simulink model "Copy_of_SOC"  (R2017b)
settings: Solver=FixedStepDiscrete  StartTime=0.0  StopTime=10.0  FixedStep=0.01  RelTol=1e-3  EnableMultiTasking=on
undefined symbols (not defined in the file): ASWTYPE_FALSE, ASWTYPE_TRUE, CaSOC_OneSOCVoltTable_mV, CaSOC_ZeroSOCTempTable_C, CaSOC_ZeroSOCVoltTable_mV, CbSOC_ManualDeplaCorrect_flg, CbSOC_ManuOCVCorrect_flg, CbSOC_SOCHighDiagOn_flg, CbSOC_SOCLowDiagOn_flg, CcSOC_ACChrgFinishDispSOC_pct, CcSOC_ACChrgFinishMaxSOC_pct, CcSOC_ACStepChrgMaxSOC_pct, CcSOC_AllowMaxCellSOC_pct, CcSOC_AllowMinCellSOC_pct, CcSOC_CapCalcCycl_ms, CcSOC_CellMinTempFilterAvg_numb, CcSOC_CellVoltMeasTol_mV, CcSOC_ChrgFishBefMaxSOC_pct, CcSOC_ChrgFishBefMinSOC_pct, CcSOC_ChrgFollowCurr_A, CcSOC_DCChrgFinishDispSOC_pct, CcSOC_DCChrgFinishMaxSOC_pct, CcSOC_DCStepChrgMaxSOC_pct, CcSOC_DeplaCellVoltMeasTol_mV, CcSOC_DeplaCorrectSOCDiff_pct, CcSOC_DisChrgFlwCurr_A, CcSOC_DispSOCChgSleepTime_min, CcSOC_DispSOCCordRunTi_ms, CcSOC_DispSOCErr_pct, CcSOC_FlwTarSOCDiff_pct, CcSOC_FullChrgTempThrld_C, CcSOC_MaxFlwDispSOC_pct, CcSOC_MinFlwDispSOC_pct, CcSOC_OCVCorrectRunTime_ms, CcSOC_OCVCorrectSleepTime_min, CcSOC_OCVCorrectSOCDiff_pct, CcSOC_OCVPeakCellVoltDev_mV, CcSOC_OCVPeakCellVoltTime_ms, CcSOC_PackSOCUseMax_pct, CcSOC_PackSOCUseMin_pct, CcSOC_SOCDeplaCurrThrd_A, CcSOC_SOCDeplaCurrThrdTi_ms, CcSOC_SOCDeplaNoOCVTi_min, CcSOC_SOCDeplaOCVTi_min, CcSOC_SOCHighAlarmThrld_pct, CcSOC_SOCHighWarningThrld_pct, CcSOC_SOCHysValue_pct, CcSOC_SOCLowAlarmThrld_pct, CcSOC_SOCLowWarningThrld_pct, CcSOC_ZeroMinSOC_pct, CcSOC_ZeroPackCrntThrd_A, CcSOC_ZeroSOCRunTime_ms, Enum_CTCCtrCtlConnMode, Enum_MSMBMUState, SOC_CONST0_NUMB, SOC_CONST1000_NUMB, SOC_CONST100_NUMB, SOC_CONST2080_NUMB, SOC_CONST3600000_NUMB, SOC_CONST60000_NUMB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
libraries: AIWAYS_Powertrain_BMS_lib x109
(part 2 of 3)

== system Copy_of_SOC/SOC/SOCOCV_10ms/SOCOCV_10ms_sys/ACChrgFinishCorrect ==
  LcCDP_MinCellAvgFitTemp_C : Inport
  Enable : EnablePort
  Constant1 : Constant  Value=CcSOC_ACChrgFinishDispSOC_pct
  Constant2 : Constant  Value=CcSOC_FullChrgTempThrld_C
  Data Store Write2 : AIWAYS_Powertrain_BMS_lib/Signals/Data Store Write  Priority=0  DSW=EcNVM_DispSOC_pct
  MaxMinSOCCorrect : Subsystem  TreatAsAtomicUnit=on
  Relational Operator : RelationalOperator  OutDataTypeStr=boolean
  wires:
  Relational Operator/1 -> MaxMinSOCCorrect/Enable
  Constant2/1 -> Relational Operator/2
  LcCDP_MinCellAvgFitTemp_C/1 -> Relational Operator/1
  Constant1/1 -> Data Store Write2/1

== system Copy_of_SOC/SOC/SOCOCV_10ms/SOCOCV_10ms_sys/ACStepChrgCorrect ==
  Enable : EnablePort
  Add : Sum  Inputs=+-  AccumDataTypeStr=single  OutDataTypeStr=single
  Add1 : Sum  Inputs=+-  AccumDataTypeStr=single  OutDataTypeStr=single
  Constant : Constant  Value=CcSOC_ACStepChrgMaxSOC_pct
  Constant1 : Constant  Value=CcSOC_ACStepChrgMaxSOC_pct
  Constant2 : Constant  Value=SOC_CONST100_NUMB
  Constant3 : Constant  Value=SOC_CONST0_NUMB
  Data Store Read : AIWAYS_Powertrain_BMS_lib/Signals/Data Store Read  Priority=0  DSR=EcNVM_MinCellSOC_pct
  Data Store Read1 : AIWAYS_Powertrain_BMS_lib/Signals/Data Store Read  Priority=0  DSR=EcNVM_MaxCellSOC_pct
  Data Store Write : AIWAYS_Powertrain_BMS_lib/Signals/Data Store Write  DSW=EcNVM_MaxCellSOC_pct
  Data Store Write1 : AIWAYS_Powertrain_BMS_lib/Signals/Data Store Write  DSW=EcNVM_MinCellSOC_pct
  Limiter : AIWAYS_Powertrain_BMS_lib/Nonlinear Blocks/Limiter
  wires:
  Constant/1 -> Data Store Write/1
  Data Store Read/1 -> Add/1
  Data Store Read1/1 -> Add1/1
  Constant1/1 -> Add1/2
  Add1/1 -> Add/2
  Limiter/1 -> Data Store Write1/1
  Constant2/1 -> Limiter/1
  Constant3/1 -> Limiter/2
  Add/1 -> Limiter/3

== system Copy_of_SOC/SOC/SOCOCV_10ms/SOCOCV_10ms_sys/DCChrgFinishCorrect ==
  LcCDP_MinCellAvgFitTemp_C : Inport
  Enable : EnablePort
  Constant1 : Constant  Value=CcSOC_DCChrgFinishDispSOC_pct
  Constant2 : Constant  Value=CcSOC_FullChrgTempThrld_C
  Data Store Write1 : AIWAYS_Powertrain_BMS_lib/Signals/Data Store Write  DSW=EcNVM_DispSOC_pct
  MaxMinSOCCorrect : Subsystem  TreatAsAtomicUnit=on
  Relational Operator : RelationalOperator  OutDataTypeStr=boolean
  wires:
  Relational Operator/1 -> MaxMinSOCCorrect/Enable
  Constant2/1 -> Relational Operator/2
  LcCDP_MinCellAvgFitTemp_C/1 -> Relational Operator/1
  Constant1/1 -> Data Store Write1/1

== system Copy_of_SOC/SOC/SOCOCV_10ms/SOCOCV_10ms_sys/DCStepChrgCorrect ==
  Enable : EnablePort
  Add : Sum  Inputs=+-  AccumDataTypeStr=single  OutDataTypeStr=single
  Add1 : Sum  Inputs=+-  AccumDataTypeStr=single  OutDataTypeStr=single
  Constant : Constant  Value=CcSOC_DCStepChrgMaxSOC_pct
  Constant1 : Constant  Value=CcSOC_DCStepChrgMaxSOC_pct
  Constant2 : Constant  Value=SOC_CONST100_NUMB
  Constant3 : Constant  Value=SOC_CONST0_NUMB
  Data Store Read : AIWAYS_Powertrain_BMS_lib/Signals/Data Store Read  Priority=0  DSR=EcNVM_MinCellSOC_pct
  Data Store Read1 : AIWAYS_Powertrain_BMS_lib/Signals/Data Store Read  Priority=0  DSR=EcNVM_MaxCellSOC_pct
  Data Store Write : AIWAYS_Powertrain_BMS_lib/Signals/Data Store Write  DSW=EcNVM_MaxCellSOC_pct
  Data Store Write1 : AIWAYS_Powertrain_BMS_lib/Signals/Data Store Write  DSW=EcNVM_MinCellSOC_pct
  Limiter : AIWAYS_Powertrain_BMS_lib/Nonlinear Blocks/Limiter
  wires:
  Limiter/1 -> Data Store Write1/1
  Add/1 -> Limiter/3
  Add1/1 -> Add/2
  Constant1/1 -> Add1/2
  Data Store Read1/1 -> Add1/1
  Data Store Read/1 -> Add/1
  Constant/1 -> Data Store Write/1
  Constant2/1 -> Limiter/1
  Constant3/1 -> Limiter/2

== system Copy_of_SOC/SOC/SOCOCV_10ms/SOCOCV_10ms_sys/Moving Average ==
  note: Moving Average
  u : Inport
  R : Inport  Port=2  OutDataTypeStr=boolean
  Chart : Stateflow chart  TreatAsAtomicUnit=on
  Signal Conversion : SignalConversion  ConversionOutput=Contiguous copy  OverrideOpt=off
  y : Outport
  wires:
  Signal Conversion/1 -> y/1
  Chart/1(Y) -> Signal Conversion/1
  u/1 -> Chart/1(u)
  R/1 -> Chart/2(R)

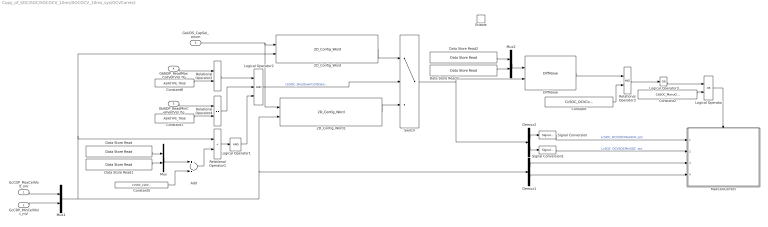
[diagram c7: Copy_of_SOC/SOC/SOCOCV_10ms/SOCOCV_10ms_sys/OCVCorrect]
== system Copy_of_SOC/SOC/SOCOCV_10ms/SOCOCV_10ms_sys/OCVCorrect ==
  GcCDP_MaxCellVolt_mV : Inport
  GcCDP_MinCellVolt_mV : Inport  Port=2
  GeUDS_CapSel_enum : Inport  Port=3
  GbNDP_ReadMaxCellVoltVld_flg : Inport  Port=4
  GbNDP_ReadMinCellVoltVld_flg : Inport  Port=5
  Enable : EnablePort
  2D_Config_Word : AIWAYS_Powertrain_BMS_lib/Signals/2D_Config_Word  Default_Cal_Breakpoint1_Name=CaSOC_CATL203ChrgOCVSOCCellVolt_mV  Default_Cal_Table1_Name=CaSOC_CATL203ChrgOCVSOCCellSOC_pct  CATL153Ah_Cal_Breakpoint1_Name=CaSOC_TFE177ChrgOCVSOCCellVolt_mV  CATL153Ah_Cal_Table1_Name=CaSOC_TFE177ChrgOCVSOCCellSOC_pct  CATL180Ah_Cal_Breakpoint1_Name=CaSOC_TFE177ChrgOCVSOCCellVolt_mV  CATL180Ah_Cal_Table1_Name=CaSOC_TFE177ChrgOCVSOCCellSOC_pct  CATL177Ah_Cal_Breakpoint1_Name=CaSOC_CATL177ChrgOCVSOCCellVolt_mV  CATL177Ah_Cal_Table1_Name=CaSOC_CATL177ChrgOCVSOCCellSOC_pct  CATL203Ah_Cal_Breakpoint1_Name=CaSOC_CATL203ChrgOCVSOCCellVolt_mV  CATL203Ah_Cal_Table1_Name=CaSOC_CATL203ChrgOCVSOCCellSOC_pct  CATL51Ah_Cal_Breakpoint1_Name=CaSOC_TFE177ChrgOCVSOCCellVolt_mV  CATL51Ah_Cal_Table1_Name=CaSOC_TFE177ChrgOCVSOCCellSOC_pct  CATL132Ah_Cal_Breakpoint1_Name=CaSOC_TFE177ChrgOCVSOCCellVolt_mV  CATL132Ah_Cal_Table1_Name=CaSOC_TFE177ChrgOCVSOCCellSOC_pct  XWD75Ah_Cal_Breakpoint1_Name=CaSOC_XWD75ChrgOCVSOCCellVolt_mV  XWD75Ah_Cal_Table1_Name=CaSOC_XWD75ChrgOCVSOCCellSOC_pct  TFE177Ah_Cal_Breakpoint1_Name=CaSOC_TFE177ChrgOCVSOCCellVolt_mV  TFE177Ah_Cal_Table1_Name=CaSOC_TFE177ChrgOCVSOCCellSOC_pct  CATLCTP248Ah_Cal_Breakpoint1_Name=CaSOC_TFE177ChrgOCVSOCCellVolt_mV  CATLCTP248Ah_Cal_Table1_Name=CaSOC_TFE177ChrgOCVSOCCellSOC_pct
  2D_Config_Word1 : AIWAYS_Powertrain_BMS_lib/Signals/2D_Config_Word  Default_Cal_Breakpoint1_Name=CaSOC_CATL203DisChrgOCVSOCCellVolt_mV  Default_Cal_Table1_Name=CaSOC_CATL203DisChrgOCVSOCCellSOC_pct  CATL153Ah_Cal_Breakpoint1_Name=CaSOC_TFE177DisChrgOCVSOCCellVolt_mV  CATL153Ah_Cal_Table1_Name=CaSOC_TFE177DisChrgOCVSOCCellSOC_pct  CATL180Ah_Cal_Breakpoint1_Name=CaSOC_TFE177DisChrgOCVSOCCellVolt_mV  CATL180Ah_Cal_Table1_Name=CaSOC_TFE177DisChrgOCVSOCCellSOC_pct  CATL177Ah_Cal_Breakpoint1_Name=CaSOC_CATL177DisChrgOCVSOCCellVolt_mV  CATL177Ah_Cal_Table1_Name=CaSOC_CATL177DisChrgOCVSOCCellSOC_pct  CATL203Ah_Cal_Breakpoint1_Name=CaSOC_CATL203DisChrgOCVSOCCellVolt_mV  CATL203Ah_Cal_Table1_Name=CaSOC_CATL203DisChrgOCVSOCCellSOC_pct  CATL51Ah_Cal_Breakpoint1_Name=CaSOC_TFE177DisChrgOCVSOCCellVolt_mV  CATL51Ah_Cal_Table1_Name=CaSOC_TFE177DisChrgOCVSOCCellSOC_pct  CATL132Ah_Cal_Breakpoint1_Name=CaSOC_TFE177DisChrgOCVSOCCellVolt_mV  CATL132Ah_Cal_Table1_Name=CaSOC_TFE177DisChrgOCVSOCCellSOC_pct  XWD75Ah_Cal_Breakpoint1_Name=CaSOC_XWD75DisChrgOCVSOCCellVolt_mV  XWD75Ah_Cal_Table1_Name=CaSOC_XWD75DisChrgOCVSOCCellSOC_pct  TFE177Ah_Cal_Breakpoint1_Name=CaSOC_TFE177DisChrgOCVSOCCellVolt_mV  TFE177Ah_Cal_Table1_Name=CaSOC_TFE177DisChrgOCVSOCCellSOC_pct  CATLCTP248Ah_Cal_Breakpoint1_Name=CaSOC_TFE177DisChrgOCVSOCCellVolt_mV  CATLCTP248Ah_Cal_Table1_Name=CaSOC_TFE177DisChrgOCVSOCCellSOC_pct
  Add : Sum  Inputs=+-  AccumDataTypeStr=uint16  OutDataTypeStr=uint16
  Constant : Constant  Value=CcSOC_OCVCorrectSOCDiff_pct
  Constant1 : Constant  Value=ASWTYPE_TRUE
  Constant2 : Constant  Value=CbSOC_ManuOCVCorrect_flg
  Constant5 : Constant  Value=CcSOC_CellVoltMeasTol_mV
  Constant6 : Constant  Value=ASWTYPE_TRUE
  Data Store Read : AIWAYS_Powertrain_BMS_lib/Signals/Data Store Read  Priority=0  DSR=EcNVM_MaxCellVolt_mV
  Data Store Read1 : AIWAYS_Powertrain_BMS_lib/Signals/Data Store Read  Priority=0  DSR=EcNVM_MinCellVolt_mV
  Data Store Read2 : AIWAYS_Powertrain_BMS_lib/Signals/Data Store Read  Priority=0  DSR=EcNVM_MaxCellSOC_pct
  Data Store Read3 : AIWAYS_Powertrain_BMS_lib/Signals/Data Store Read  Priority=0  DSR=EcNVM_MinCellSOC_pct
  Demux1 : Demux  Outputs=2
  Demux2 : Demux  Outputs=2
  DiffValue : AIWAYS_Powertrain_BMS_lib/Mathematical Functions/DiffValue
  Logical Operator : Logic  Operator=OR  AllPortsSameDT=off  OutDataTypeStr=boolean
  Logical Operator1 : Logic  Inputs=1  AllPortsSameDT=off  OutDataTypeStr=boolean
  Logical Operator2 : Logic  Inputs=3  AllPortsSameDT=off  OutDataTypeStr=boolean
  Logical Operator3 : Logic  Operator=OR  Inputs=1  AllPortsSameDT=off  OutDataTypeStr=boolean
  MaxCellCorrect : Subsystem  TreatAsAtomicUnit=on
  Mux : Mux  Inputs=2
  Mux1 : Mux  Inputs=2
  Mux2 : Mux  Inputs=2
  Relational Operator1 : RelationalOperator  Operator=<  OutDataTypeStr=boolean
  Relational Operator2 : RelationalOperator  Operator===  OutDataTypeStr=boolean
  Relational Operator3 : RelationalOperator  OutDataTypeStr=boolean
  Relational Operator4 : RelationalOperator  Operator===  OutDataTypeStr=boolean
  Signal Conversion : SignalConversion  OverrideOpt=off
  Signal Conversion1 : SignalConversion  OverrideOpt=off
  Switch : Switch  Criteria=u2 ~= 0
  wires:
  Logical Operator3/1 -> Logical Operator/1
  Constant2/1 -> Logical Operator/2
  Signal Conversion/1 -> MaxCellCorrect/1(LcSOC_OCVSOCMaxSOC_pct)  "LcSOC_OCVSOCMaxSOC_pct"
  Logical Operator/1 -> MaxCellCorrect/Enable
  Relational Operator3/1 -> Logical Operator3/1
  Data Store Read1/1 -> Mux/2
  Data Store Read/1 -> Mux/1
  GcCDP_MinCellVolt_mV/1 -> Mux1/2
  GcCDP_MaxCellVolt_mV/1 -> Mux1/1
  Mux1/1 -> 2D_Config_Word/2, Relational Operator1/1, 2D_Config_Word1/2, Demux1/1
  Relational Operator1/1 -> Logical Operator1/1
  Mux/1 -> Add/1
  Constant5/1 -> Add/2
  Constant6/1 -> Relational Operator2/2
  GbNDP_ReadMaxCellVoltVld_flg/1 -> Relational Operator2/1
  GbNDP_ReadMinCellVoltVld_flg/1 -> Relational Operator4/1
  Constant1/1 -> Relational Operator4/2
  Relational Operator2/1 -> Logical Operator2/1
  Relational Operator4/1 -> Logical Operator2/2
  Add/1 -> Relational Operator1/2
  Data Store Read2/1 -> Mux2/1
  Data Store Read3/1 -> Mux2/2
  DiffValue/1 -> Relational Operator3/1
  Constant/1 -> Relational Operator3/2
  Mux2/1 -> DiffValue/1
  Demux2/1 -> Signal Conversion/1
  Demux2/2 -> Signal Conversion1/1
  Signal Conversion1/1 -> MaxCellCorrect/2(LcSOC_OCVSOCMinSOC_pct)  "LcSOC_OCVSOCMinSOC_pct"
  Logical Operator2/1 -> Switch/2  "LbSOC_ShutdownCellState_flg"
  2D_Config_Word/1 -> Switch/1
  2D_Config_Word1/1 -> Switch/3
  Switch/1 -> DiffValue/2, Demux2/1
  Logical Operator1/1 -> Logical Operator2/3
  Demux1/1 -> MaxCellCorrect/3(GcCDP_MaxCellVolt_mV)
  Demux1/2 -> MaxCellCorrect/4(GcCDP_MinCellVolt_mV)
  GeUDS_CapSel_enum/1 -> 2D_Config_Word1/1, 2D_Config_Word/1

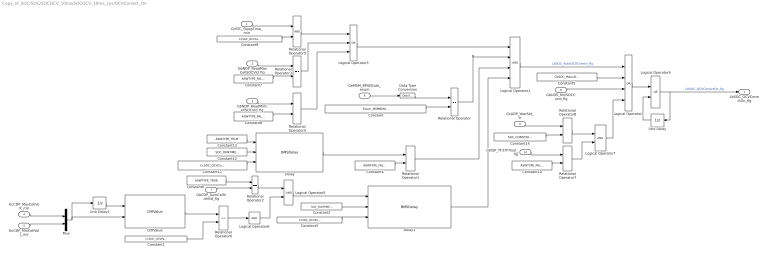
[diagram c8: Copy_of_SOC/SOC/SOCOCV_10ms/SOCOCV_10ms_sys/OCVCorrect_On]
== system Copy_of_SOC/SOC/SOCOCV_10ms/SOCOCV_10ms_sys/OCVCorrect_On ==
  GcRTC_SleepTime_min : Inport
  GbNDP_ReadMaxCellSOCVld_flg : Inport  Port=2
  GbNDP_ReadMinCellSOCVld_flg : Inport  Port=3
  GcCDP_MaxCellVolt_mV : Inport  Port=4
  GcCDP_MinCellVolt_mV : Inport  Port=5
  GeMSM_BMUState_enum : Inport  Port=6
  GbCDP_SumCellVoltVld_flg : Inport  Port=7
  GbUDS_MnlSOCCorrd_flg : Inport  Port=8
  GcADP_YearSet_Yr : Inport  Port=9
  GbISP_TF37FTiout_flg : Inport  Port=10
  Constant : Constant  Value=Enum_MSMBMUState.Enum_MSMBMUState_Standby
  Constant1 : Constant  Value=CcSOC_OCVPeakCellVoltDev_mV
  Constant{4,7..8,10} (4 alike) : Constant  Value=ASWTYPE_FALSE
  Constant11 : Constant  Value=CcSOC_OCVCorrectRunTime_ms
  Constant12 : Constant  Value=SOC_RUNTIME_MS
  Constant13 : Constant  Value=ASWTYPE_TRUE
  Constant14 : Constant  Value=SOC_CONST2080_NUMB
  Constant2 : Constant  Value=SOC_RUNTIME_MS
  Constant3 : Constant  Value=CcSOC_OCVPeakCellVoltTime_ms
  Constant5 : Constant  Value=CbSOC_ManuOCVCorrect_flg
  Constant6 : Constant  Value=ASWTYPE_TRUE
  Constant9 : Constant  Value=CcSOC_OCVCorrectSleepTime_min
  Data Type Conversion : DataTypeConversion
  Delay : AIWAYS_Powertrain_BMS_lib/Debounce & Delay/BMSDelay
  Delay1 : AIWAYS_Powertrain_BMS_lib/Debounce & Delay/BMSDelay
  DiffValue : AIWAYS_Powertrain_BMS_lib/Mathematical Functions/DiffValue
  Logical Operator1 : Logic  Inputs=4  AllPortsSameDT=off  OutDataTypeStr=boolean
  Logical Operator2 : Logic  Operator=OR  Inputs=4  AllPortsSameDT=off  OutDataTypeStr=boolean
  Logical Operator3 : Logic  Operator=OR  Inputs=3  AllPortsSameDT=off  OutDataTypeStr=boolean
  Logical Operator4 : Logic  Operator=OR  AllPortsSameDT=off  OutDataTypeStr=boolean
  Logical Operator5 : Logic  AllPortsSameDT=off  OutDataTypeStr=boolean
  Logical Operator6 : Logic  Inputs=1  AllPortsSameDT=off  OutDataTypeStr=boolean
  Logical Operator7 : Logic  AllPortsSameDT=off  OutDataTypeStr=boolean
  Mux : Mux  Inputs=2
  Relational Operator{,1..4,7..8} (7 alike) : RelationalOperator  Operator===  OutDataTypeStr=boolean
  Relational Operator5 : RelationalOperator  OutDataTypeStr=boolean
  Relational Operator6 : RelationalOperator  Operator=<=  OutDataTypeStr=boolean
  Unit Delay : UnitDelay  SampleTime=-1  StateName=StateName
  Unit Delay1 : UnitDelay  SampleTime=-1  StateName=StateName
  LbSOC_OCVCorrectOn_flg : Outport
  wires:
  Constant12/1 -> Delay/2
  Relational Operator6/1 -> Logical Operator6/1
  Delay/1 -> Relational Operator1/1
  Constant7/1 -> Relational Operator3/2
  Logical Operator6/1 -> Logical Operator5/2
  Mux/1 -> Unit Delay1/1, DiffValue/2
  GbNDP_ReadMinCellSOCVld_flg/1 -> Relational Operator4/1
  Constant9/1 -> Relational Operator5/2
  Constant1/1 -> Relational Operator6/2
  Logical Operator4/1 -> LbSOC_OCVCorrectOn_flg/1, Unit Delay/1  "LbSOC_OCVCorrectOn_flg"
  Logical Operator5/1 -> Delay1/1
  Data Type Conversion/1 -> Relational Operator/1
  GcCDP_MaxCellVolt_mV/1 -> Mux/1
  Relational Operator4/1 -> Logical Operator3/3
  Logical Operator2/1 -> Logical Operator4/1
  Constant6/1 -> Relational Operator2/1
  GbUDS_MnlSOCCorrd_flg/1 -> Logical Operator2/3
  GbNDP_ReadMaxCellSOCVld_flg/1 -> Relational Operator3/1
  Constant3/1 -> Delay1/3
  GcCDP_MinCellVolt_mV/1 -> Mux/2
  Constant2/1 -> Delay1/2
  DiffValue/1 -> Relational Operator6/1
  Constant/1 -> Relational Operator/2
  Constant13/1 -> Delay/1
  Relational Operator3/1 -> Logical Operator3/2
  GcRTC_SleepTime_min/1 -> Relational Operator5/1
  Unit Delay/1 -> Logical Operator4/2
  Constant8/1 -> Relational Operator4/2
  GbCDP_SumCellVoltVld_flg/1 -> Relational Operator2/2
  Relational Operator5/1 -> Logical Operator3/1
  Constant11/1 -> Delay/3
  Unit Delay1/1 -> DiffValue/1
  Relational Operator2/1 -> Logical Operator5/1
  GeMSM_BMUState_enum/1 -> Data Type Conversion/1
  Logical Operator1/1 -> Logical Operator2/1  "LbSOC_AutoOCVCorrect_flg"
  Constant5/1 -> Logical Operator2/2
  Constant4/1 -> Relational Operator1/2
  Relational Operator/1 -> Logical Operator1/2
  Relational Operator1/1 -> Logical Operator1/3
  Delay1/1 -> Logical Operator1/4
  Logical Operator3/1 -> Logical Operator1/1
  Constant10/1 -> Relational Operator7/2
  GbISP_TF37FTiout_flg/1 -> Relational Operator7/1
  Constant14/1 -> Relational Operator8/2
  GcADP_YearSet_Yr/1 -> Relational Operator8/1
  Relational Operator8/1 -> Logical Operator7/1
  Relational Operator7/1 -> Logical Operator7/2
  Logical Operator7/1 -> Logical Operator2/4

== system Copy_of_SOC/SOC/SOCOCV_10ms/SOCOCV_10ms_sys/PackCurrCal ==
  GcHDP_PackCrnt_A : Inport
  Add : Sum  OutDataTypeStr=Inherit: Inherit via back propagation
  Add2 : Sum  AccumDataTypeStr=single  OutDataTypeStr=single
  Constant : Constant  Value=SOC_CONST0_NUMB
  Constant1 : Constant  Value=SOC_CONST0_NUMB
  Constant2 : Constant  Value=CcSOC_CapCalcCycl_ms
  Constant5 : Constant  Value=SOC_RUNTIME_MS
  Data Type Conversion1 : DataTypeConversion
  PackCurrAvg : Subsystem
  Relational Operator : RelationalOperator  OutDataTypeStr=boolean
  Switch : Switch  Criteria=u2 ~= 0
  Switch1 : Switch  Criteria=u2 ~= 0
  Unit Delay : UnitDelay  SampleTime=-1  StateName=StateName
  Unit Delay1 : UnitDelay  SampleTime=-1  StateName=StateName
  LcSOC_PackCurrAvg_A : Outport
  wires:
  Unit Delay/1 -> Add2/1
  PackCurrAvg/1(LcSOC_PackCurrAvg_A) -> LcSOC_PackCurrAvg_A/1
  Switch/1 -> Unit Delay/1
  Add2/1 -> PackCurrAvg/1(LcSOC_SumPackCurr_A), Switch/3
  GcHDP_PackCrnt_A/1 -> Add2/2
  Add/1 -> Switch1/3, Relational Operator/1
  Relational Operator/1 -> Switch/2, PackCurrAvg/Enable, Switch1/2  "LbSOC_CapCalcCycl_flg"
  Unit Delay1/1 -> Add/1
  Constant2/1 -> Relational Operator/2
  Constant5/1 -> Add/2
  Switch1/1 -> Unit Delay1/1
  Constant1/1 -> Data Type Conversion1/1
  Constant/1 -> Switch/1
  Data Type Conversion1/1 -> Switch1/1

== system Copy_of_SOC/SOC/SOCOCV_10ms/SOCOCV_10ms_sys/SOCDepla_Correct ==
  GcHDP_PackCrnt_A : Inport
  GbHDP_PackCrntVld_flg : Inport  Port=2
  GcCDP_MaxCellVolt_mV : Inport  Port=3
  GcCDP_MinCellVolt_mV : Inport  Port=4
  GbCDP_SumCellVoltVld_flg : Inport  Port=5
  GcRTC_SleepTime_min : Inport  Port=6
  GeUDS_CapSel_enum : Inport  Port=7
  LbSOC_OCVCorrectOn_flg : Inport  Port=8
  Bus Creator1 : BusCreator  Inputs=7
  Bus Selector1 : BusSelector  OutputSignals=LbSOC_OCVCorrectOn_flg,GcCDP_MaxCellVolt_mV,GcCDP_MinCellVolt_mV,GbCDP_SumCellVoltVld_flg,GeUDS_CapSel_enum
  Bus Selector2 : BusSelector  OutputSignals=GcHDP_PackCrnt_A,GbHDP_PackCrntVld_flg,LbSOC_OCVCorrectOn_flg
  Bus Selector5 : BusSelector  OutputSignals=GcCDP_MaxCellVolt_mV,GcCDP_MinCellVolt_mV,GbCDP_SumCellVoltVld_flg
  CellDeplaState_Judge : Subsystem  TreatAsAtomicUnit=on
  CellDeplaTiCond_Judge : Subsystem
  CellDeplaTi_Cal : Subsystem
  SOC_GcSOC_CellDeplaTi_min : AIWAYS_Powertrain_BMS_lib/Signals/OverWrite  OverWrite_Value=CcSOC_CellDeplaTiOvr_min  OverWrite_flag=CbSOC_CellDeplaTiOvrSwt_flg
  Unit Delay : UnitDelay  SampleTime=-1  StateName=StateName
  GcSOC_CellDeplaTi_min : Outport
  GbSOC_SOCDeplaTiReach_flg : Outport  Port=2
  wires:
  GcHDP_PackCrnt_A/1 -> Bus Creator1/1  "GcHDP_PackCrnt_A"
  GbHDP_PackCrntVld_flg/1 -> Bus Creator1/2  "GbHDP_PackCrntVld_flg"
  GcCDP_MaxCellVolt_mV/1 -> Bus Creator1/3  "GcCDP_MaxCellVolt_mV"
  GcCDP_MinCellVolt_mV/1 -> Bus Creator1/4  "GcCDP_MinCellVolt_mV"
  Bus Selector5/1 -> CellDeplaState_Judge/1(GcCDP_MaxCellVolt_mV)  "<GcCDP_MaxCellVolt_mV>"
  Bus Selector5/2 -> CellDeplaState_Judge/2(GcCDP_MinCellVolt_mV)  "<GcCDP_MinCellVolt_mV>"
  LbSOC_OCVCorrectOn_flg/1 -> Bus Creator1/6  "LbSOC_OCVCorrectOn_flg"
  GbCDP_SumCellVoltVld_flg/1 -> Bus Creator1/5  "GbCDP_SumCellVoltVld_flg"
  Bus Selector5/3 -> CellDeplaState_Judge/3(GbCDP_SumCellVoltVld_flg)  "<GbCDP_SumCellVoltVld_flg>"
  Bus Creator1/1 -> Bus Selector2/1, Bus Selector5/1, Bus Selector1/1
  GcRTC_SleepTime_min/1 -> CellDeplaTi_Cal/2(GcRTC_SleepTime_min)  "GcRTC_SleepTime_min"
  CellDeplaState_Judge/1(LbSOC_DeplaCellVoltChrgState_flg) -> CellDeplaTiCond_Judge/2(LbSOC_DeplaCellVoltChrgState_flg)
  CellDeplaTi_Cal/1(GcSOC_CellDeplaTi_min) -> SOC_GcSOC_CellDeplaTi_min/1
  Bus Selector1/1 -> CellDeplaTiCond_Judge/3(LbSOC_OCVCorrectOn_flg)  "<LbSOC_OCVCorrectOn_flg>"
  Bus Selector1/2 -> CellDeplaTiCond_Judge/4(GcCDP_MaxCellVolt_mV)  "<GcCDP_MaxCellVolt_mV>"
  Bus Selector1/3 -> CellDeplaTiCond_Judge/5(GcCDP_MinCellVolt_mV)  "<GcCDP_MinCellVolt_mV>"
  CellDeplaTi_Cal/2(LbSOC_CellDeplaCond_flg) -> CellDeplaState_Judge/Enable
  Unit Delay/1 -> CellDeplaTi_Cal/1(GbSOC_SOCDeplaTiReach_flg)
  SOC_GcSOC_CellDeplaTi_min/1 -> CellDeplaTiCond_Judge/1(GcSOC_CellDeplaTi_min), GcSOC_CellDeplaTi_min/1  "GcSOC_CellDeplaTi_min"
  CellDeplaTiCond_Judge/1(GbSOC_SOCDeplaTiReach_flg) -> GbSOC_SOCDeplaTiReach_flg/1, Unit Delay/1
  Bus Selector2/1 -> CellDeplaTi_Cal/3(GcHDP_PackCrnt_A)  "<GcHDP_PackCrnt_A>"
  Bus Selector2/3 -> CellDeplaTi_Cal/5(LbSOC_OCVCorrectOn_flg)  "<LbSOC_OCVCorrectOn_flg>"
  Bus Selector2/2 -> CellDeplaTi_Cal/4(GbHDP_PackCrntVld_flg)  "<GbHDP_PackCrntVld_flg>"
  Bus Selector1/4 -> CellDeplaTiCond_Judge/6(GbCDP_SumCellVoltVld_flg)  "<GbCDP_SumCellVoltVld_flg>"
  GeUDS_CapSel_enum/1 -> Bus Creator1/7  "GeUDS_CapSel_enum"
  Bus Selector1/5 -> CellDeplaTiCond_Judge/7(GeUDS_CapSel_enum)  "<GeUDS_CapSel_enum>"

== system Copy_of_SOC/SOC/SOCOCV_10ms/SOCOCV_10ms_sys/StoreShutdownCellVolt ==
  GcCDP_MaxCellVolt_mV : Inport
  GcCDP_MinCellVolt_mV : Inport  Port=2
  Enable : EnablePort
  Data Store Write : AIWAYS_Powertrain_BMS_lib/Signals/Data Store Write  DSW=EcNVM_MaxCellVolt_mV
  Data Store Write1 : AIWAYS_Powertrain_BMS_lib/Signals/Data Store Write  DSW=EcNVM_MinCellVolt_mV
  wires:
  GcCDP_MaxCellVolt_mV/1 -> Data Store Write/1
  GcCDP_MinCellVolt_mV/1 -> Data Store Write1/1

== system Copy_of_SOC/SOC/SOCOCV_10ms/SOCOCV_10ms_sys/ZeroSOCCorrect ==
  Enable : EnablePort  StatesWhenEnabling=reset
  Add : Sum  Inputs=+-  AccumDataTypeStr=single  OutDataTypeStr=single
  Add1 : Sum  AccumDataTypeStr=single  OutDataTypeStr=single
  Constant{1..2,4..5} (4 alike) : Constant  Value=SOC_CONST0_NUMB
  Constant3 : Constant  Value=SOC_CONST100_NUMB
  Data Store Read : AIWAYS_Powertrain_BMS_lib/Signals/Data Store Read  Priority=0  DSR=EcNVM_MinCellSOC_pct
  Data Store Read1 : AIWAYS_Powertrain_BMS_lib/Signals/Data Store Read  Priority=0  DSR=EcNVM_MaxCellSOC_pct
  Data Store Write : AIWAYS_Powertrain_BMS_lib/Signals/Data Store Write  DSW=EcNVM_MinCellSOC_pct
  Data Store Write1 : AIWAYS_Powertrain_BMS_lib/Signals/Data Store Write  DSW=EcNVM_MaxCellSOC_pct
  Data Store Write2 : AIWAYS_Powertrain_BMS_lib/Signals/Data Store Write  Priority=0  DSW=EcNVM_DispSOC_pct
  Limiter : AIWAYS_Powertrain_BMS_lib/Nonlinear Blocks/Limiter
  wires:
  Constant1/1 -> Data Store Write2/1
  Limiter/1 -> Data Store Write1/1
  Constant4/1 -> Limiter/2
  Constant3/1 -> Limiter/1
  Data Store Read1/1 -> Add/1
  Constant5/1 -> Data Store Write/1
  Data Store Read/1 -> Add/2
  Add/1 -> Add1/1
  Add1/1 -> Limiter/3
  Constant2/1 -> Add1/2

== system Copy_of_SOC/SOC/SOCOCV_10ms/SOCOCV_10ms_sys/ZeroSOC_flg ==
  GcCDP_MinCellVolt_mV : Inport
  GcHDP_PackCrnt_A : Inport  Port=2
  LcCDP_MinCellAvgFitTemp_C : Inport  Port=3
  1-D Lookup Table1 : Lookup_n-D  NumberOfTableDimensions=1  BreakpointsForDimension1=CaSOC_ZeroSOCTempTable_C  Table=CaSOC_ZeroSOCVoltTable_mV  ExtrapMethod=Clip  UseLastTableValue=on  InternalRulePriority=Speed  OutDataTypeStr=Inherit: Inherit from 'Table data'  RndMeth=Simplest
  1-D Lookup Table2 : Lookup_n-D  NumberOfTableDimensions=1  BreakpointsForDimension1=CaSOC_ZeroSOCTempTable_C  Table=CaSOC_OneSOCVoltTable_mV  ExtrapMethod=Clip  UseLastTableValue=on  InternalRulePriority=Speed  OutDataTypeStr=Inherit: Inherit from 'Table data'  RndMeth=Simplest
  Abs : Abs
  BMSDelay : AIWAYS_Powertrain_BMS_lib/Debounce & Delay/BMSDelay
  BMSDelay1 : AIWAYS_Powertrain_BMS_lib/Debounce & Delay/BMSDelay
  Constant1 : Constant  Value=CcSOC_ZeroPackCrntThrd_A
  Constant11 : Constant  Value=CcSOC_ZeroSOCRunTime_ms
  Constant12 : Constant  Value=SOC_RUNTIME_MS
  Constant2 : Constant  Value=SOC_RUNTIME_MS
  Constant3 : Constant  Value=CcSOC_ZeroSOCRunTime_ms
  Constant4 : Constant  Value=ASWTYPE_FALSE
  Constant7 : Constant  Value=ASWTYPE_TRUE
  Data Type Conversion3 : DataTypeConversion  OutDataTypeStr=fixdt(0,8,1,-40)  RndMeth=Round
  Logical : Logic  OutDataTypeStr=boolean
  Relational Operator1 : RelationalOperator  Operator=<=  OutDataTypeStr=boolean
  Relational Operator2 : RelationalOperator  Operator=<=  OutDataTypeStr=boolean
  Relational Operator3 : RelationalOperator  Operator=<=  OutDataTypeStr=boolean
  Switch : Switch  Criteria=u2 ~= 0  Threshold=1  RndMeth=Zero
  Switch1 : Switch  Criteria=u2 ~= 0  Threshold=1  RndMeth=Zero
  Unit Delay21 : UnitDelay  SampleTime=-1  StateName=StateName
  LbSOC_ZeroSOCCorrect_flg : Outport
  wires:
  GcCDP_MinCellVolt_mV/1 -> Relational Operator3/2, Relational Operator2/1
  LcCDP_MinCellAvgFitTemp_C/1 -> Data Type Conversion3/1
  1-D Lookup Table1/1 -> Relational Operator2/2
  Constant12/1 -> BMSDelay/2
  Constant11/1 -> BMSDelay/3
  Data Type Conversion3/1 -> 1-D Lookup Table2/1, 1-D Lookup Table1/1
  GcHDP_PackCrnt_A/1 -> Abs/1
  Constant1/1 -> Relational Operator1/2
  Relational Operator2/1 -> Logical/1
  Relational Operator1/1 -> Logical/2
  Abs/1 -> Relational Operator1/1
  Logical/1 -> BMSDelay/1
  Switch/1 -> Unit Delay21/1, LbSOC_ZeroSOCCorrect_flg/1  "LbSOC_ZeroSOCCorrect_flg"
  BMSDelay/1 -> Switch1/2  "LbSOC_ZeroSOCReach_flg"
  Constant7/1 -> Switch1/1
  Switch1/1 -> Switch/3
  1-D Lookup Table2/1 -> Relational Operator3/1
  Relational Operator3/1 -> BMSDelay1/1
  Constant2/1 -> BMSDelay1/2
  Constant3/1 -> BMSDelay1/3
  BMSDelay1/1 -> Switch/2  "LbSOC_OneSOCReach_flg"
  Constant4/1 -> Switch/1
  Unit Delay21/1 -> Switch1/3

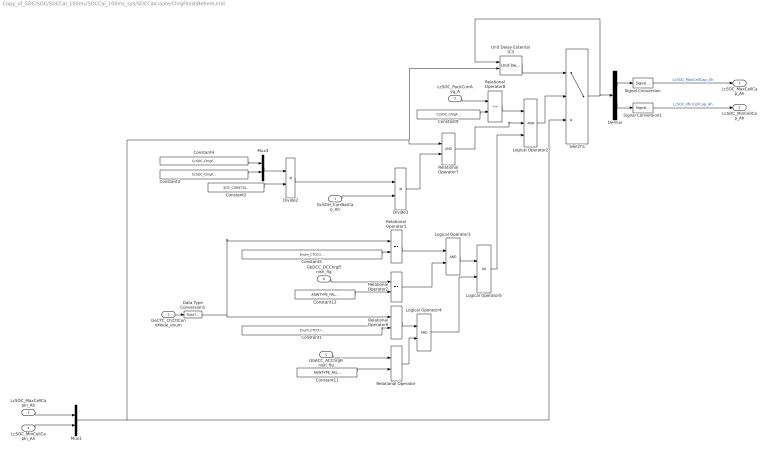
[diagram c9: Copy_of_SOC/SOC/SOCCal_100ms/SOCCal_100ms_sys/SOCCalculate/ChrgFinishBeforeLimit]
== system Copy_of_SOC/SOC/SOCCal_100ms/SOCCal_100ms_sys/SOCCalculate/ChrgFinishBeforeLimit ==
  GcSOH_CurrBatCap_Ah : Inport
  GeCTC_CtrCtlConnMode_enum : Inport  Port=2
  LcSOC_MaxCellCapIn_Ah : Inport  Port=3
  LcSOC_MinCellCapIn_Ah : Inport  Port=4
  GbACC_ACChrgFinish_flg : Inport  Port=5
  GbDCC_DCChrgFinish_flg : Inport  Port=6
  LcSOC_PackCurrAvg_A : Inport  Port=7
  Constant1 : Constant  Value=Enum_CTCCtrCtlConnMode.Enum_CTCCtrCtlConnMode_ACChrg
  Constant11 : Constant  Value=ASWTYPE_FALSE
  Constant13 : Constant  Value=ASWTYPE_FALSE
  Constant2 : Constant  Value=SOC_CONST100_NUMB
  Constant3 : Constant  Value=CcSOC_ChrgFishBefMinSOC_pct
  Constant4 : Constant  Value=CcSOC_ChrgFishBefMaxSOC_pct
  Constant5 : Constant  Value=Enum_CTCCtrCtlConnMode.Enum_CTCCtrCtlConnMode_DCChrg
  Constant9 : Constant  Value=CcSOC_ChrgFollowCurr_A
  Data Type Conversion1 : DataTypeConversion
  Demux : Demux  Outputs=2
  Divide2 : Product  Inputs=*/  OutDataTypeStr=single
  Divide3 : Product  Inputs=**  OutDataTypeStr=single
  Logical Operator2 : Logic  Inputs=3  AllPortsSameDT=off  OutDataTypeStr=boolean
  Logical Operator3 : Logic  AllPortsSameDT=off  OutDataTypeStr=boolean
  Logical Operator4 : Logic  AllPortsSameDT=off  OutDataTypeStr=boolean
  Logical Operator5 : Logic  Operator=OR  AllPortsSameDT=off  OutDataTypeStr=boolean
  Mux1 : Mux  Inputs=2
  Mux3 : Mux  Inputs=2
  Relational Operator{,1..2,6} (4 alike) : RelationalOperator  Operator===  OutDataTypeStr=boolean
  Relational Operator7 : RelationalOperator  OutDataTypeStr=boolean
  Relational Operator8 : RelationalOperator  Operator=<=  OutDataTypeStr=boolean
  Signal Conversion : SignalConversion  OverrideOpt=off
  Signal Conversion1 : SignalConversion  OverrideOpt=off
  Switch1 : Switch  Criteria=u2 ~= 0
  Unit Delay External IC3 : AIWAYS_Powertrain_BMS_lib/Delay Blocks/Unit Delay External IC
  LcSOC_MaxCellCap_Ah : Outport
  LcSOC_MinCellCap_Ah : Outport  Port=2
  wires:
  Unit Delay External IC3/1 -> Switch1/1
  Relational Operator7/1 -> Logical Operator2/2
  Relational Operator8/1 -> Logical Operator2/1
  Divide3/1 -> Relational Operator7/2
  Constant11/1 -> Relational Operator/2
  Demux/1 -> Signal Conversion/1
  Demux/2 -> Signal Conversion1/1
  LcSOC_MaxCellCapIn_Ah/1 -> Mux1/1
  LcSOC_MinCellCapIn_Ah/1 -> Mux1/2
  GbACC_ACChrgFinish_flg/1 -> Relational Operator/1
  Signal Conversion/1 -> LcSOC_MaxCellCap_Ah/1  "LcSOC_MaxCellCap_Ah"
  Signal Conversion1/1 -> LcSOC_MinCellCap_Ah/1  "LcSOC_MinCellCap_Ah"
  GcSOH_CurrBatCap_Ah/1 -> Divide3/2
  Constant4/1 -> Mux3/1
  Constant3/1 -> Mux3/2
  Mux3/1 -> Divide2/1
  Divide2/1 -> Divide3/1
  Constant2/1 -> Divide2/2
  Constant13/1 -> Relational Operator2/2
  GbDCC_DCChrgFinish_flg/1 -> Relational Operator2/1
  Logical Operator2/1 -> Switch1/2
  Switch1/1 -> Demux/1, Unit Delay External IC3/1
  Mux1/1 -> Unit Delay External IC3/2, Relational Operator7/1, Switch1/3
  GeCTC_CtrCtlConnMode_enum/1 -> Data Type Conversion1/1
  Relational Operator2/1 -> Logical Operator3/2
  Constant1/1 -> Relational Operator6/2
  Relational Operator6/1 -> Logical Operator4/1
  Relational Operator/1 -> Logical Operator4/2
  Logical Operator3/1 -> Logical Operator5/1
  Logical Operator4/1 -> Logical Operator5/2
  Logical Operator5/1 -> Logical Operator2/3
  Constant9/1 -> Relational Operator8/2
  LcSOC_PackCurrAvg_A/1 -> Relational Operator8/1
  Constant5/1 -> Relational Operator1/2
  Data Type Conversion1/1 -> Relational Operator1/1, Relational Operator6/1
  Relational Operator1/1 -> Logical Operator3/1

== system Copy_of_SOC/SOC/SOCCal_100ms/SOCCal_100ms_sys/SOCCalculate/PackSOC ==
  GcSOC_MaxCellSOC_pct : Inport
  GcSOC_MinCellSOC_pct : Inport  Port=2
  Add1 : Sum  Inputs=+-  OutDataTypeStr=Inherit: Inherit via back propagation
  Add9 : Sum  OutDataTypeStr=Inherit: Inherit via back propagation
  Bus Creator : BusCreator  Inputs=2
  Bus Selector : BusSelector  OutputSignals=LcSOC_MapMinSOC_pct
  Bus Selector1 : BusSelector  OutputSignals=LcSOC_MapMaxSOC_pct
  Bus Selector2 : BusSelector  OutputSignals=LcSOC_MapMinSOC_pct
  Bus Selector3 : BusSelector  OutputSignals=LcSOC_MapMaxSOC_pct
  Bus Selector4 : BusSelector  OutputSignals=LcSOC_MapMinSOC_pct
  Comparison1 : RelationalOperator  Operator=<  OutDataTypeStr=boolean
  Comparison2 : RelationalOperator  Operator=>  OutDataTypeStr=boolean
  Constant18 : Constant  Value=SOC_CONST100_NUMB
  Constant2 : Constant  Value=SOC_CONST100_NUMB
  Constant5 : Constant  Value=SOC_CONST100_NUMB
  Constant6 : Constant  Value=CcSOC_PackSOCUseMax_pct
  Constant7 : Constant  Value=CcSOC_PackSOCUseMin_pct
  Constant8 : Constant  Value=SOC_CONST0_NUMB
  GcSOC_PackSOC_pctOverWrite : AIWAYS_Powertrain_BMS_lib/Signals/OverWrite  OverWrite_Value=CcSOC_PackSOCOvr_pct  OverWrite_flag=CbSOC_PackSOCOvrSwt_flg
  Limiter : AIWAYS_Powertrain_BMS_lib/Nonlinear Blocks/Limiter
  Product2 : Product  OutDataTypeStr=Inherit: Inherit via back propagation
  Protected Division2 : AIWAYS_Powertrain_BMS_lib/Arithmetic Operators/Protected Division
  Signal Conversion : SignalConversion  ConversionOutput=Contiguous copy  OverrideOpt=off
  Signal Conversion1 : SignalConversion  ConversionOutput=Contiguous copy  OverrideOpt=off
  Switch : Switch  Criteria=u2 ~= 0  Threshold=1  RndMeth=Zero
  Switch1 : Switch  Criteria=u2 ~= 0  Threshold=1  RndMeth=Zero
  GcSOC_PackSOC_pct : Outport
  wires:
  GcSOC_PackSOC_pctOverWrite/1 -> GcSOC_PackSOC_pct/1  "GcSOC_PackSOC_pct"
  Constant5/1 -> Limiter/1
  Constant8/1 -> Limiter/2
  Limiter/1 -> GcSOC_PackSOC_pctOverWrite/1
  Constant6/1 -> Comparison2/2
  Comparison2/1 -> Switch/2
  Switch/1 -> Switch1/3
  Comparison1/1 -> Switch1/2
  Constant7/1 -> Comparison1/2
  Switch1/1 -> Limiter/3
  GcSOC_MaxCellSOC_pct/1 -> Signal Conversion1/1
  GcSOC_MinCellSOC_pct/1 -> Signal Conversion/1
  Add9/1 -> Protected Division2/2
  Signal Conversion1/1 -> Bus Creator/2  "LcSOC_MapMaxSOC_pct"
  Signal Conversion/1 -> Bus Creator/1  "LcSOC_MapMinSOC_pct"
  Constant2/1 -> Add1/1
  Bus Selector/1 -> Protected Division2/1  "<LcSOC_MapMinSOC_pct>"
  Add1/1 -> Add9/2
  Bus Selector1/1 -> Add1/2  "<LcSOC_MapMaxSOC_pct>"
  Bus Selector2/1 -> Add9/1  "<LcSOC_MapMinSOC_pct>"
  Bus Creator/1 -> Bus Selector4/1, Bus Selector3/1, Bus Selector/1, Bus Selector2/1, Bus Selector1/1
  Bus Selector3/1 -> Switch/1, Comparison2/1  "<LcSOC_MapMaxSOC_pct>"
  Bus Selector4/1 -> Switch1/1, Comparison1/1  "<LcSOC_MapMinSOC_pct>"
  Protected Division2/1 -> Product2/1
  Constant18/1 -> Product2/2
  Product2/1 -> Switch/3  "LcSOC_MapPackSOC_pct"

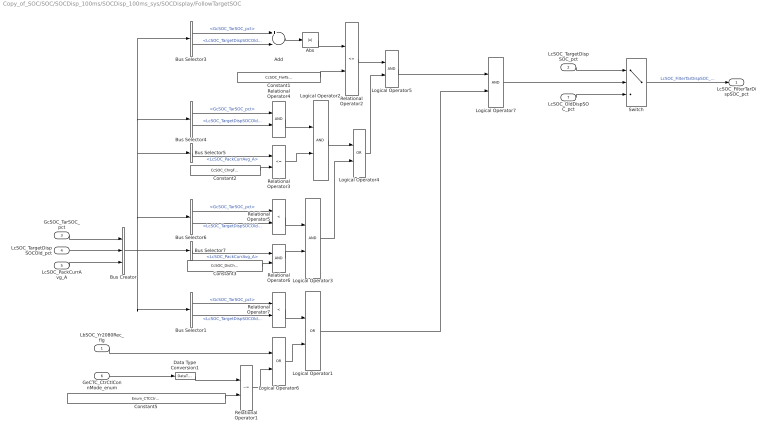
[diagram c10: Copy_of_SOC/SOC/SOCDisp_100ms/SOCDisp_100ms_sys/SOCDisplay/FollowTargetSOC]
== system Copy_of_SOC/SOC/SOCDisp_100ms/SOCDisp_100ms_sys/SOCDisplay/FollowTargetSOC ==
  LbSOC_Yr2080Rec_flg : Inport
  LcSOC_TargetDispSOC_pct : Inport  Port=2
  GcSOC_TarSOC_pct : Inport  Port=3
  LcSOC_TargetDispSOCOld_pct : Inport  Port=4
  LcSOC_PackCurrAvg_A : Inport  Port=5
  GeCTC_CtrCtlConnMode_enum : Inport  Port=6
  LcSOC_OldDispSOC_pct : Inport  Port=7
  Abs : Abs
  Add : Sum  Inputs=+-  OutDataTypeStr=Inherit: Inherit via back propagation
  Bus Creator : BusCreator  Inputs=3
  Bus Selector{1,3..4,6} (4 alike) : BusSelector  OutputSignals=GcSOC_TarSOC_pct,LcSOC_TargetDispSOCOld_pct
  Bus Selector5 : BusSelector  OutputSignals=LcSOC_PackCurrAvg_A
  Bus Selector7 : BusSelector  OutputSignals=LcSOC_PackCurrAvg_A
  Constant1 : Constant  Value=CcSOC_FlwTarSOCDiff_pct
  Constant2 : Constant  Value=CcSOC_ChrgFollowCurr_A
  Constant3 : Constant  Value=CcSOC_DisChrgFlwCurr_A
  Constant5 : Constant  Value=Enum_CTCCtrCtlConnMode.Enum_CTCCtrCtlConnMode_Drive
  Data Type Conversion1 : DataTypeConversion
  Logical Operator1 : Logic  Operator=OR  AllPortsSameDT=off  OutDataTypeStr=boolean
  Logical Operator{2..3,5,7} (4 alike) : Logic  AllPortsSameDT=off  OutDataTypeStr=boolean
  Logical Operator4 : Logic  Operator=OR  AllPortsSameDT=off  OutDataTypeStr=boolean
  Logical Operator6 : Logic  Operator=OR  AllPortsSameDT=off  OutDataTypeStr=boolean
  Relational Operator1 : RelationalOperator  Operator=~=  OutDataTypeStr=boolean
  Relational Operator2 : RelationalOperator  Operator=<=  OutDataTypeStr=boolean
  Relational Operator3 : RelationalOperator  Operator=<=  OutDataTypeStr=boolean
  Relational Operator4 : RelationalOperator  OutDataTypeStr=boolean
  Relational Operator5 : RelationalOperator  Operator=<  OutDataTypeStr=boolean
  Relational Operator6 : RelationalOperator  OutDataTypeStr=boolean
  Relational Operator7 : RelationalOperator  Operator=<  OutDataTypeStr=boolean
  Switch : Switch  Criteria=u2 ~= 0
  LcSOC_FilterTarDispSOC_pct : Outport
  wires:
  Bus Selector3/2 -> Add/2  "<LcSOC_TargetDispSOCOld_pct>"
  Constant3/1 -> Relational Operator6/2
  Logical Operator2/1 -> Logical Operator4/1
  Relational Operator5/1 -> Logical Operator3/1
  Relational Operator6/1 -> Logical Operator3/2
  Relational Operator2/1 -> Logical Operator5/1
  Logical Operator4/1 -> Logical Operator5/2
  Logical Operator3/1 -> Logical Operator4/2
  Switch/1 -> LcSOC_FilterTarDispSOC_pct/1  "LcSOC_FilterTarDispSOC_pct"
  LcSOC_OldDispSOC_pct/1 -> Switch/3
  Add/1 -> Abs/1
  Bus Selector3/1 -> Add/1  "<GcSOC_TarSOC_pct>"
  Constant1/1 -> Relational Operator2/2
  Relational Operator3/1 -> Logical Operator2/2
  Bus Selector6/2 -> Relational Operator5/2  "<LcSOC_TargetDispSOCOld_pct>"
  Relational Operator4/1 -> Logical Operator2/1
  Bus Selector7/1 -> Relational Operator6/1  "<LcSOC_PackCurrAvg_A>"
  Bus Selector4/1 -> Relational Operator4/1  "<GcSOC_TarSOC_pct>"
  Bus Selector4/2 -> Relational Operator4/2  "<LcSOC_TargetDispSOCOld_pct>"
  Constant2/1 -> Relational Operator3/2
  Bus Selector6/1 -> Relational Operator5/1  "<GcSOC_TarSOC_pct>"
  Bus Selector5/1 -> Relational Operator3/1  "<LcSOC_PackCurrAvg_A>"
  Abs/1 -> Relational Operator2/1
  LcSOC_TargetDispSOCOld_pct/1 -> Bus Creator/2
  GcSOC_TarSOC_pct/1 -> Bus Creator/1
  LcSOC_PackCurrAvg_A/1 -> Bus Creator/3
  LcSOC_TargetDispSOC_pct/1 -> Switch/1
  GeCTC_CtrCtlConnMode_enum/1 -> Data Type Conversion1/1
  Constant5/1 -> Relational Operator1/2
  Data Type Conversion1/1 -> Relational Operator1/1
  LbSOC_Yr2080Rec_flg/1 -> Logical Operator6/1
  Relational Operator1/1 -> Logical Operator6/2
  Bus Selector1/1 -> Relational Operator7/1  "<GcSOC_TarSOC_pct>"
  Bus Selector1/2 -> Relational Operator7/2  "<LcSOC_TargetDispSOCOld_pct>"
  Logical Operator1/1 -> Logical Operator7/2
  Relational Operator7/1 -> Logical Operator1/1
  Bus Creator/1 -> Bus Selector1/1, Bus Selector6/1, Bus Selector3/1, Bus Selector4/1, Bus Selector5/1, Bus Selector7/1
  Logical Operator5/1 -> Logical Operator7/1
  Logical Operator7/1 -> Switch/2
  Logical Operator6/1 -> Logical Operator1/2

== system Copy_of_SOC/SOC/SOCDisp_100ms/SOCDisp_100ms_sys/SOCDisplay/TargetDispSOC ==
  GcSOC_PackSOC_pct : Inport
  LcCDP_MinCellAvgFitTemp_C : Inport  Port=2
  GeUDS_CapSel_enum : Inport  Port=3
  2D_Config_Word : AIWAYS_Powertrain_BMS_lib/Signals/2D_Config_Word  Default_Cal_Breakpoint1_Name=CaSOC_TFE177TargetSOCCellTemp_C  Default_Cal_Table1_Name=CaSOC_TFE177TargetMinSOC_pct  CATL153Ah_Cal_Breakpoint1_Name=CaSOC_TFE177TargetSOCCellTemp_C  CATL153Ah_Cal_Table1_Name=CaSOC_TFE177TargetMinSOC_pct  CATL180Ah_Cal_Breakpoint1_Name=CaSOC_TFE177TargetSOCCellTemp_C  CATL180Ah_Cal_Table1_Name=CaSOC_TFE177TargetMinSOC_pct  CATL177Ah_Cal_Breakpoint1_Name=CaSOC_CATL177TargetSOCCellTemp_C  CATL177Ah_Cal_Table1_Name=CaSOC_CATL177TargetMinSOC_pct  CATL203Ah_Cal_Breakpoint1_Name=CaSOC_CATL203TargetSOCCellTemp_C  CATL203Ah_Cal_Table1_Name=CaSOC_CATL203TargetMinSOC_pct  CATL51Ah_Cal_Breakpoint1_Name=CaSOC_TFE177TargetSOCCellTemp_C  CATL51Ah_Cal_Table1_Name=CaSOC_TFE177TargetMinSOC_pct  CATL132Ah_Cal_Breakpoint1_Name=CaSOC_TFE177TargetSOCCellTemp_C  CATL132Ah_Cal_Table1_Name=CaSOC_TFE177TargetMinSOC_pct  XWD75Ah_Cal_Breakpoint1_Name=CaSOC_XWD75TargetSOCCellTemp_C  XWD75Ah_Cal_Table1_Name=CaSOC_XWD75TargetMinSOC_pct  TFE177Ah_Cal_Breakpoint1_Name=CaSOC_TFE177TargetSOCCellTemp_C  TFE177Ah_Cal_Table1_Name=CaSOC_TFE177TargetMinSOC_pct  CATLCTP248Ah_Cal_Breakpoint1_Name=CaSOC_TFE177TargetSOCCellTemp_C  CATLCTP248Ah_Cal_Table1_Name=CaSOC_TFE177TargetMinSOC_pct
  Bus Creator : BusCreator  Inputs=2
  Bus Selector : BusSelector  OutputSignals=GcSOC_PackSOC_pct
  Bus Selector1 : BusSelector  OutputSignals=LcSOC_TargetMinSOC_pct
  Bus Selector2 : BusSelector  OutputSignals=LcSOC_TargetMinSOC_pct
  Constant : Constant  Value=SOC_CONST100_NUMB
  Constant1 : Constant  Value=CcSOC_AllowMinCellSOC_pct
  Constant11 : Constant  Value=CcSOC_AllowMaxCellSOC_pct
  Constant18 : Constant  Value=SOC_CONST100_NUMB
  Constant2 : Constant  Value=SOC_CONST0_NUMB
  Data Type Conversion3 : DataTypeConversion  OutDataTypeStr=fixdt(0,8,5,-40)  RndMeth=Round
  GcSOC_TarSOC_pctOverWrite : AIWAYS_Powertrain_BMS_lib/Signals/OverWrite  OverWrite_Value=CcSOC_TarSOCOvr_pct  OverWrite_flag=CbSOC_TarSOCOvrSwt_flg
  Limiter : AIWAYS_Powertrain_BMS_lib/Nonlinear Blocks/Limiter
  MinMax1 : MinMax  Function=max  Inputs=2  OutDataTypeStr=Inherit: Inherit via back propagation  RndMeth=Zero
  Product2 : Product  OutDataTypeStr=Inherit: Inherit via back propagation
  Protected Division2 : AIWAYS_Powertrain_BMS_lib/Arithmetic Operators/Protected Division
  Sum1 : Sum  Inputs=+-  OutDataTypeStr=Inherit: Inherit via back propagation  RndMeth=Zero
  Sum2 : Sum  Inputs=+-  OutDataTypeStr=Inherit: Inherit via back propagation  RndMeth=Zero
  GcSOC_TarSOC_pct : Outport
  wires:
  GcSOC_TarSOC_pctOverWrite/1 -> GcSOC_TarSOC_pct/1  "GcSOC_TarSOC_pct"
  Constant11/1 -> Sum2/1
  Constant2/1 -> Limiter/2
  Constant/1 -> Limiter/1
  Limiter/1 -> GcSOC_TarSOC_pctOverWrite/1
  Data Type Conversion3/1 -> 2D_Config_Word/2
  GcSOC_PackSOC_pct/1 -> Bus Creator/1
  Bus Creator/1 -> Bus Selector1/1, Bus Selector/1, Bus Selector2/1
  Bus Selector/1 -> Sum1/1  "<GcSOC_PackSOC_pct>"
  Bus Selector1/1 -> Sum1/2  "<LcSOC_TargetMinSOC_pct>"
  Bus Selector2/1 -> Sum2/2  "<LcSOC_TargetMinSOC_pct>"
  Protected Division2/1 -> Product2/1
  Constant18/1 -> Product2/2
  Sum1/1 -> Protected Division2/1
  Sum2/1 -> Protected Division2/2
  2D_Config_Word/1 -> MinMax1/1
  Constant1/1 -> MinMax1/2
  MinMax1/1 -> Bus Creator/2  "LcSOC_TargetMinSOC_pct"
  Product2/1 -> Limiter/3
  LcCDP_MinCellAvgFitTemp_C/1 -> Data Type Conversion3/1
  GeUDS_CapSel_enum/1 -> 2D_Config_Word/1

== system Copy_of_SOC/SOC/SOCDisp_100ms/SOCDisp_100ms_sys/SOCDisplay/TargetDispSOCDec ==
  GcSOC_TarSOC_pct : Inport
  LcSOC_TargetDispSOCOld_pct : Inport  Port=2
  Add : Sum  Inputs=+-
  Add1 : Sum  Inputs=+-
  Add2 : Sum  Inputs=+-
  Add4 : Sum
  Constant1 : Constant  Value=CcSOC_MinFlwDispSOC_pct
  Constant2 : Constant  Value=CcSOC_MinFlwDispSOC_pct
  Data Store Read : AIWAYS_Powertrain_BMS_lib/Signals/Data Store Read  Priority=0  DSR=EcNVM_DispSOC_pct
  Divide : Product  Inputs=**
  Protected Division : AIWAYS_Powertrain_BMS_lib/Arithmetic Operators/Protected Division
  LcSOC_TargetDispSOCDec_pct : Outport
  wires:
  GcSOC_TarSOC_pct/1 -> Add/1
  Add/1 -> Divide/1
  Data Store Read/1 -> Add4/2, Add1/1
  Constant1/1 -> Add1/2
  Add1/1 -> Divide/2
  Divide/1 -> Protected Division/1
  Constant2/1 -> Add2/2
  Add2/1 -> Protected Division/2
  LcSOC_TargetDispSOCOld_pct/1 -> Add/2, Add2/1
  Protected Division/1 -> Add4/1
  Add4/1 -> LcSOC_TargetDispSOCDec_pct/1  "LcSOC_TargetDispSOCDec_pct"

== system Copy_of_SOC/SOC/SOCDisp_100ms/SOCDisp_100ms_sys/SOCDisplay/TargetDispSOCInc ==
  GcSOC_TarSOC_pct : Inport
  LcSOC_TargetDispSOCOld_pct : Inport  Port=2
  Add4 : Sum  Inputs=+-
  Add5 : Sum  Inputs=-+
  Add6 : Sum  Inputs=-+
  Add7 : Sum
  Constant2 : Constant  Value=CcSOC_MaxFlwDispSOC_pct
  Constant3 : Constant  Value=CcSOC_MaxFlwDispSOC_pct
  Data Store Read1 : AIWAYS_Powertrain_BMS_lib/Signals/Data Store Read  Priority=0  DSR=EcNVM_DispSOC_pct
  Divide2 : Product  Inputs=**
  Protected Division : AIWAYS_Powertrain_BMS_lib/Arithmetic Operators/Protected Division
  LcSOC_TargetDispSOCInc_pct : Outport
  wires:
  GcSOC_TarSOC_pct/1 -> Add4/1
  Add4/1 -> Divide2/1
  Data Store Read1/1 -> Add5/1, Add7/2
  Constant2/1 -> Add5/2
  Add5/1 -> Divide2/2
  Divide2/1 -> Protected Division/1
  Constant3/1 -> Add6/2
  Add6/1 -> Protected Division/2
  LcSOC_TargetDispSOCOld_pct/1 -> Add4/2, Add6/1
  Protected Division/1 -> Add7/1
  Add7/1 -> LcSOC_TargetDispSOCInc_pct/1  "LcSOC_TargetDispSOCInc_pct"

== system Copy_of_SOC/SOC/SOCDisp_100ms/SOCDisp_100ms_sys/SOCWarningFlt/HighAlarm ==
  GcSOC_DispSOC_pct : Inport
  Constant : Constant  Value=CcSOC_SOCHighAlarmThrld_pct
  Constant1 : Constant  Value=CcSOC_SOCHysValue_pct
  Constant2 : Constant  Value=CbSOC_SOCHighDiagOn_flg
  Logical Operator : Logic  AllPortsSameDT=off  OutDataTypeStr=boolean
  Relational Operator : RelationalOperator
  SOC_GbSOC_SOCHghAlrm_flg : AIWAYS_Powertrain_BMS_lib/Signals/OverWrite  OverWrite_Value=CbSOC_SOCHghAlrmOvr_flg  OverWrite_flag=CbSOC_SOCHghAlrmOvrSwt_flg
  Sum : Sum  OutDataTypeStr=Inherit: Inherit via back propagation
  GbSOC_SOCHghAlrm_flg : Outport
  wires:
  Constant1/1 -> Sum/2
  Constant/1 -> Sum/1
  GcSOC_DispSOC_pct/1 -> Relational Operator/1
  Sum/1 -> Relational Operator/2
  SOC_GbSOC_SOCHghAlrm_flg/1 -> GbSOC_SOCHghAlrm_flg/1  "GbSOC_SOCHghAlrm_flg"
  Constant2/1 -> Logical Operator/2
  Relational Operator/1 -> Logical Operator/1
  Logical Operator/1 -> SOC_GbSOC_SOCHghAlrm_flg/1

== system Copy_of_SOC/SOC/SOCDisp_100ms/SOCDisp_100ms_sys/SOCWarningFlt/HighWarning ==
  GcSOC_DispSOC_pct : Inport
  Constant : Constant  Value=CcSOC_SOCHighWarningThrld_pct
  Constant1 : Constant  Value=CcSOC_SOCHysValue_pct
  Constant2 : Constant  Value=CbSOC_SOCHighDiagOn_flg
  Logical Operator : Logic  AllPortsSameDT=off  OutDataTypeStr=boolean
  Relational Operator : RelationalOperator
  SOC_GbSOC_SOCHghWarn_flg : AIWAYS_Powertrain_BMS_lib/Signals/OverWrite  OverWrite_Value=CbSOC_SOCHghWarnOvr_flg  OverWrite_flag=CbSOC_SOCHghWarnOvrSwt_flg
  Sum : Sum  OutDataTypeStr=Inherit: Inherit via back propagation
  GbSOC_SOCHghWarn_flg : Outport
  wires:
  Sum/1 -> Relational Operator/2
  GcSOC_DispSOC_pct/1 -> Relational Operator/1
  Constant/1 -> Sum/1
  Constant1/1 -> Sum/2
  Relational Operator/1 -> Logical Operator/1
  Constant2/1 -> Logical Operator/2
  SOC_GbSOC_SOCHghWarn_flg/1 -> GbSOC_SOCHghWarn_flg/1  "GbSOC_SOCHghWarn_flg"
  Logical Operator/1 -> SOC_GbSOC_SOCHghWarn_flg/1

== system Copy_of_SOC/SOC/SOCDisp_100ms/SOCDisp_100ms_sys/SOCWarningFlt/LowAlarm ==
  GcSOC_DispSOC_pct : Inport
  Constant2 : Constant  Value=CbSOC_SOCLowDiagOn_flg
  Constant5 : Constant  Value=CcSOC_SOCLowAlarmThrld_pct
  Constant6 : Constant  Value=CcSOC_SOCHysValue_pct
  Logical Operator : Logic  AllPortsSameDT=off  OutDataTypeStr=boolean
  Relational Operator1 : RelationalOperator  Operator=<=
  SOC_GbSOC_SOCLowAlrm_flg : AIWAYS_Powertrain_BMS_lib/Signals/OverWrite  OverWrite_Value=CbSOC_SOCLowAlrmOvr_flg  OverWrite_flag=CbSOC_SOCLowAlrmOvrSwt_flg
  Sum1 : Sum  Inputs=+-  OutDataTypeStr=Inherit: Inherit via back propagation
  GbSOC_SOCLowAlrm_flg : Outport
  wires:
  GcSOC_DispSOC_pct/1 -> Relational Operator1/1
  SOC_GbSOC_SOCLowAlrm_flg/1 -> GbSOC_SOCLowAlrm_flg/1  "GbSOC_SOCLowAlrm_flg"
  Constant2/1 -> Logical Operator/2
  Relational Operator1/1 -> Logical Operator/1
  Logical Operator/1 -> SOC_GbSOC_SOCLowAlrm_flg/1
  Constant6/1 -> Sum1/2
  Constant5/1 -> Sum1/1
  Sum1/1 -> Relational Operator1/2

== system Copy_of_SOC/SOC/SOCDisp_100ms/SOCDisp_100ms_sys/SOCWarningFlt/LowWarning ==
  GcSOC_DispSOC_pct : Inport
  Constant2 : Constant  Value=CbSOC_SOCLowDiagOn_flg
  Constant5 : Constant  Value=CcSOC_SOCLowWarningThrld_pct
  Constant6 : Constant  Value=CcSOC_SOCHysValue_pct
  Logical Operator : Logic  AllPortsSameDT=off  OutDataTypeStr=boolean
  Relational Operator1 : RelationalOperator  Operator=<=
  SOC_GbSOC_SOCLowWarn_flg : AIWAYS_Powertrain_BMS_lib/Signals/OverWrite  OverWrite_Value=CbSOC_SOCLowWarnOvr_flg  OverWrite_flag=CbSOC_SOCLowWarnOvrSwt_flg
  Sum1 : Sum  Inputs=+-  OutDataTypeStr=Inherit: Inherit via back propagation
  GbSOC_SOCLowWarn_flg : Outport
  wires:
  GcSOC_DispSOC_pct/1 -> Relational Operator1/1
  Constant2/1 -> Logical Operator/2
  Relational Operator1/1 -> Logical Operator/1
  SOC_GbSOC_SOCLowWarn_flg/1 -> GbSOC_SOCLowWarn_flg/1  "GbSOC_SOCLowWarn_flg"
  Logical Operator/1 -> SOC_GbSOC_SOCLowWarn_flg/1
  Constant5/1 -> Sum1/1
  Sum1/1 -> Relational Operator1/2
  Constant6/1 -> Sum1/2

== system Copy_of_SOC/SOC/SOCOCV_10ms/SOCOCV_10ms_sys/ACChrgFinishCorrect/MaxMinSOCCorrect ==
  Enable : EnablePort
  Add : Sum  Inputs=+-  AccumDataTypeStr=single  OutDataTypeStr=single
  Add1 : Sum  Inputs=+-  AccumDataTypeStr=single  OutDataTypeStr=single
  Constant : Constant  Value=CcSOC_ACChrgFinishMaxSOC_pct
  Constant1 : Constant  Value=CcSOC_ACChrgFinishMaxSOC_pct
  Constant2 : Constant  Value=SOC_CONST100_NUMB
  Constant3 : Constant  Value=SOC_CONST0_NUMB
  Data Store Read : AIWAYS_Powertrain_BMS_lib/Signals/Data Store Read  Priority=0  DSR=EcNVM_MinCellSOC_pct
  Data Store Read1 : AIWAYS_Powertrain_BMS_lib/Signals/Data Store Read  Priority=0  DSR=EcNVM_MaxCellSOC_pct
  Data Store Write : AIWAYS_Powertrain_BMS_lib/Signals/Data Store Write  DSW=EcNVM_MaxCellSOC_pct
  Data Store Write1 : AIWAYS_Powertrain_BMS_lib/Signals/Data Store Write  DSW=EcNVM_MinCellSOC_pct
  Limiter : AIWAYS_Powertrain_BMS_lib/Nonlinear Blocks/Limiter
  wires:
  Limiter/1 -> Data Store Write1/1
  Add/1 -> Limiter/3
  Add1/1 -> Add/2
  Constant1/1 -> Add1/2
  Data Store Read1/1 -> Add1/1
  Data Store Read/1 -> Add/1
  Constant/1 -> Data Store Write/1
  Constant3/1 -> Limiter/2
  Constant2/1 -> Limiter/1

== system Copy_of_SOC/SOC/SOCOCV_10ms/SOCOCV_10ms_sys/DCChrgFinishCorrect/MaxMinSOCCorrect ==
  Enable : EnablePort
  Add : Sum  Inputs=+-  AccumDataTypeStr=single  OutDataTypeStr=single
  Add1 : Sum  Inputs=+-  AccumDataTypeStr=single  OutDataTypeStr=single
  Constant : Constant  Value=CcSOC_DCChrgFinishMaxSOC_pct
  Constant1 : Constant  Value=CcSOC_DCChrgFinishMaxSOC_pct
  Constant2 : Constant  Value=SOC_CONST100_NUMB
  Constant3 : Constant  Value=SOC_CONST0_NUMB
  Data Store Read : AIWAYS_Powertrain_BMS_lib/Signals/Data Store Read  Priority=0  DSR=EcNVM_MinCellSOC_pct
  Data Store Read1 : AIWAYS_Powertrain_BMS_lib/Signals/Data Store Read  Priority=0  DSR=EcNVM_MaxCellSOC_pct
  Data Store Write : AIWAYS_Powertrain_BMS_lib/Signals/Data Store Write  DSW=EcNVM_MaxCellSOC_pct
  Data Store Write1 : AIWAYS_Powertrain_BMS_lib/Signals/Data Store Write  DSW=EcNVM_MinCellSOC_pct
  Limiter : AIWAYS_Powertrain_BMS_lib/Nonlinear Blocks/Limiter
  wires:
  Limiter/1 -> Data Store Write1/1
  Add/1 -> Limiter/3
  Add1/1 -> Add/2
  Constant1/1 -> Add1/2
  Data Store Read1/1 -> Add1/1
  Data Store Read/1 -> Add/1
  Constant/1 -> Data Store Write/1
  Constant3/1 -> Limiter/2
  Constant2/1 -> Limiter/1
